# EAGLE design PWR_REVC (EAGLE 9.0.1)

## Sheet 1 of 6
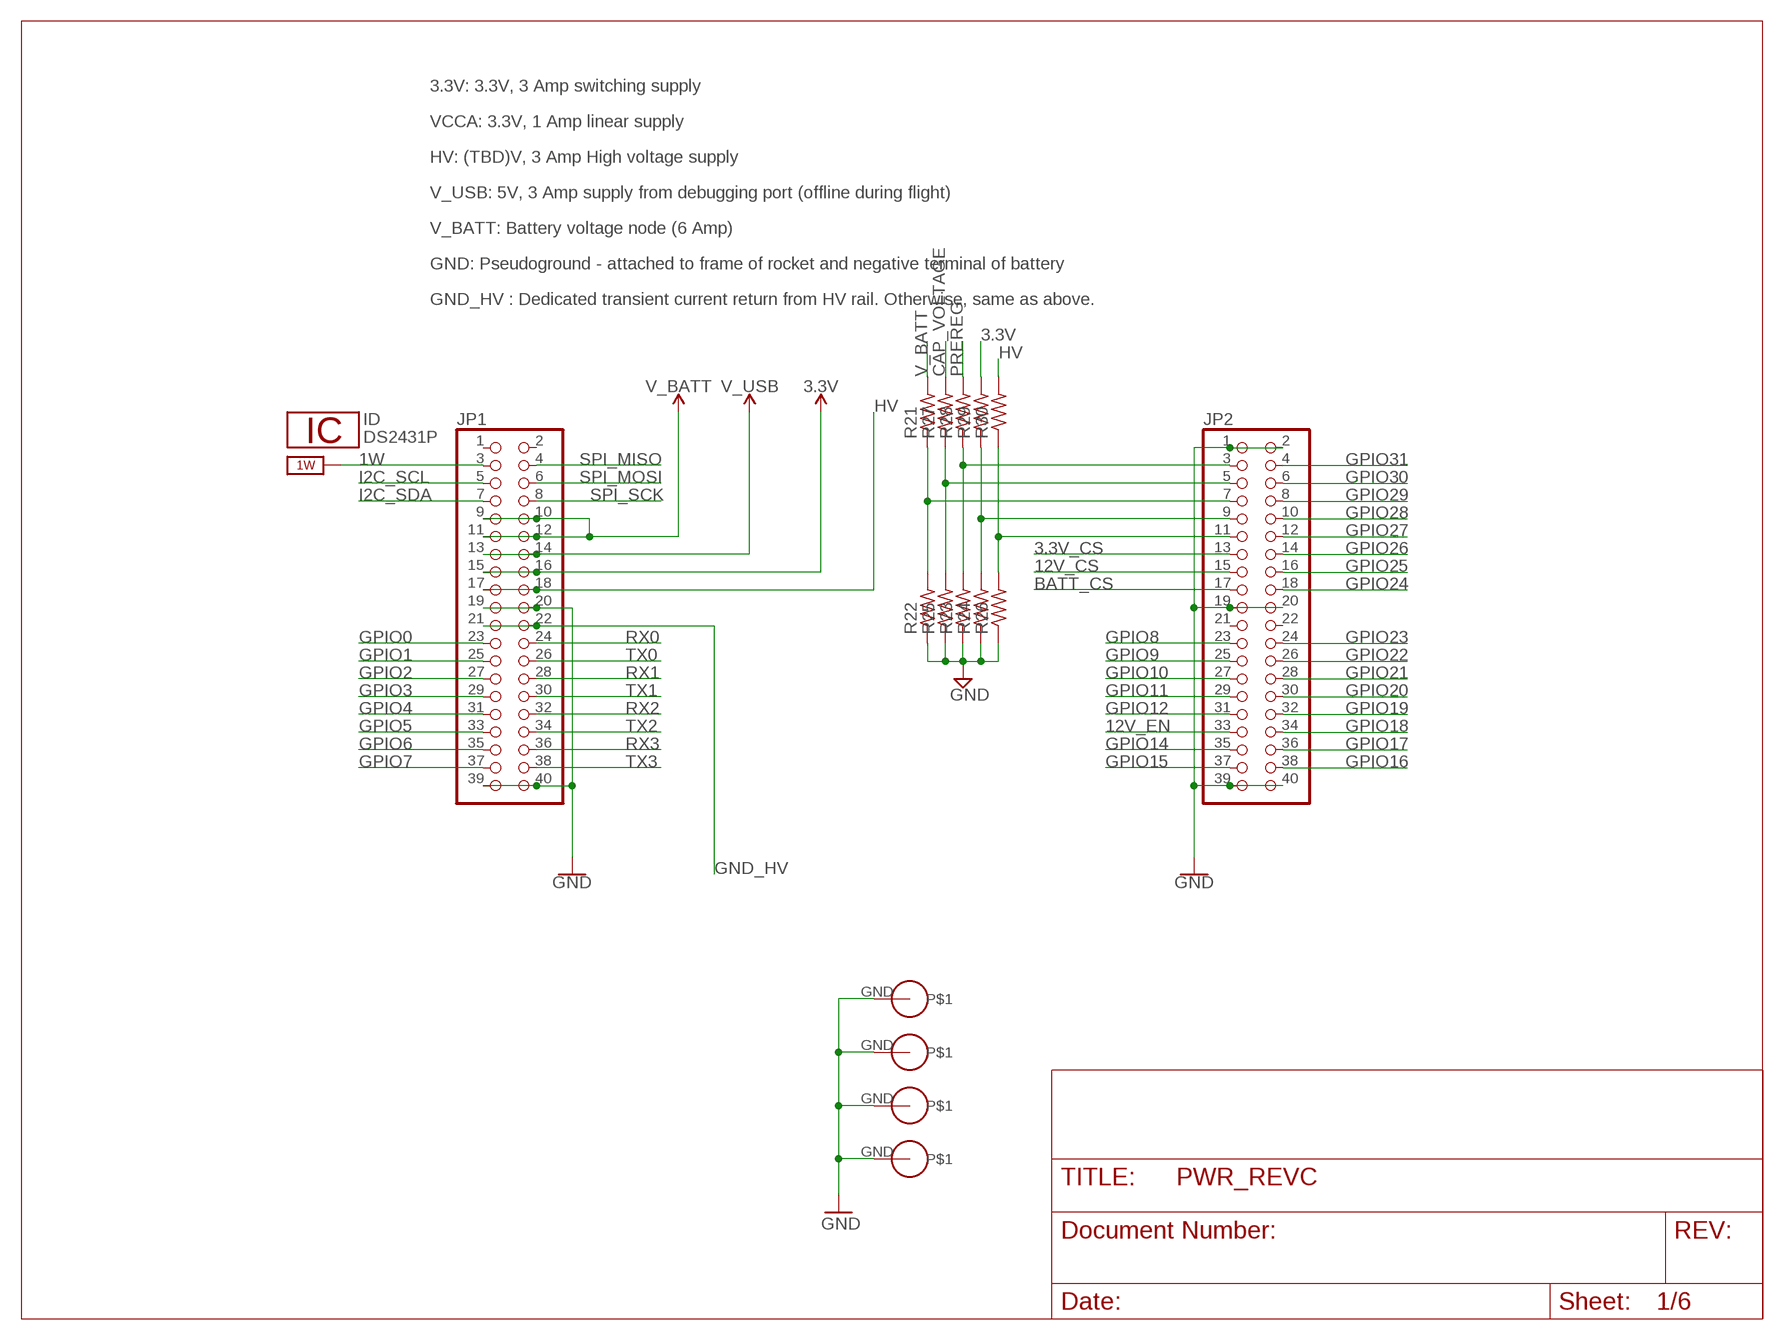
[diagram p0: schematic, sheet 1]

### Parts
ID  DS2431P  [TSOC6]
JP1  PINHD-2X20  [2X20]
JP2  PINHD-2X20  [2X20]
R21  R-US_R1206  [R1206]
R22  R-US_R1206  [R1206]
R23  R-US_R1206  [R1206]
R24  R-US_R1206  [R1206]
R25  R-US_R1206  [R1206]
R26  R-US_R1206  [R1206]
R27  R-US_R1206  [R1206]
R28  R-US_R1206  [R1206]
R29  R-US_R1206  [R1206]
R30  R-US_R1206  [R1206]
U$1  PS/104-MOUNTING-HOLE  [PC/104-MOUNTING-HOLE]
U$2  PS/104-MOUNTING-HOLE  [PC/104-MOUNTING-HOLE]
U$3  PS/104-MOUNTING-HOLE  [PC/104-MOUNTING-HOLE]
U$4  PS/104-MOUNTING-HOLE  [PC/104-MOUNTING-HOLE]

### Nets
1W: JP1.3 ; supply symbol labelled 1W_SUP
3.3V: JP1.15 JP1.16 R29.2 ; also sheet 2,6
3.3V_CS: JP2.13 ; also sheet 6
12V_CS: JP2.15 ; also sheet 6
12V_EN: JP2.33 ; also sheet 4
BATT_CS: JP2.17 ; also sheet 6
CAP_VOLTAGE: R27.2 ; also sheet 5
GND: JP1.19 JP1.20 JP1.39 JP1.40 JP2.1 JP2.2 JP2.19 JP2.20 JP2.39 JP2.40 R22.1 R23.1 R24.1 R25.1 R26.1 U$1.GND U$2.GND U$3.GND U$4.GND ; also sheet 2,3,4,5,6
GND_HV: JP1.21 JP1.22 ; also sheet 4
GPIO0: JP1.23
GPIO1: JP1.25
GPIO2: JP1.27
GPIO3: JP1.29
GPIO4: JP1.31
GPIO5: JP1.33
GPIO6: JP1.35
GPIO7: JP1.37
GPIO8: JP2.23
GPIO9: JP2.25
GPIO10: JP2.27
GPIO11: JP2.29
GPIO12: JP2.31
GPIO14: JP2.35
GPIO15: JP2.37
GPIO16: JP2.38
GPIO17: JP2.36
GPIO18: JP2.34
GPIO19: JP2.32
GPIO20: JP2.30
GPIO21: JP2.28
GPIO22: JP2.26
GPIO23: JP2.24
GPIO24: JP2.18
GPIO25: JP2.16
GPIO26: JP2.14
GPIO27: JP2.12
GPIO28: JP2.10
GPIO29: JP2.8
GPIO30: JP2.6
GPIO31: JP2.4
HV: JP1.17 JP1.18 R30.2 ; also sheet 4,6
I2C_SCL: JP1.5
I2C_SDA: JP1.7
N$28: JP2.7 R21.1 R22.2
N$30: JP2.5 R25.2 R27.1
N$31: JP2.3 R23.2 R28.1
N$32: JP2.9 R24.2 R29.1
N$33: JP2.11 R26.2 R30.1
PREREG: R28.2 ; also sheet 2,3,4,5
RX0: JP1.24
RX1: JP1.28
RX2: JP1.32
RX3: JP1.36
SPI_MISO: JP1.4
SPI_MOSI: JP1.6
SPI_SCK: JP1.8
TX0: JP1.26
TX1: JP1.30
TX2: JP1.34
TX3: JP1.38
V_BATT: JP1.9 JP1.10 JP1.11 JP1.12 R21.2 ; also sheet 3,6
V_USB: JP1.13 JP1.14
Unconnected: JP1.1 JP1.2 JP2.21 JP2.22

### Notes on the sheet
- 3.3V: 3.3V, 3 Amp switching supply
- VCCA: 3.3V, 1 Amp linear supply
- HV: (TBD)V, 3 Amp High voltage supply
- V_USB: 5V, 3 Amp supply from debugging port (offline during flight)
- V_BATT: Battery voltage node (6 Amp)
- GND: Pseudoground - attached to frame of rocket and negative terminal of battery
- GND_HV : Dedicated transient current return from HV rail. Otherwise, same as above.

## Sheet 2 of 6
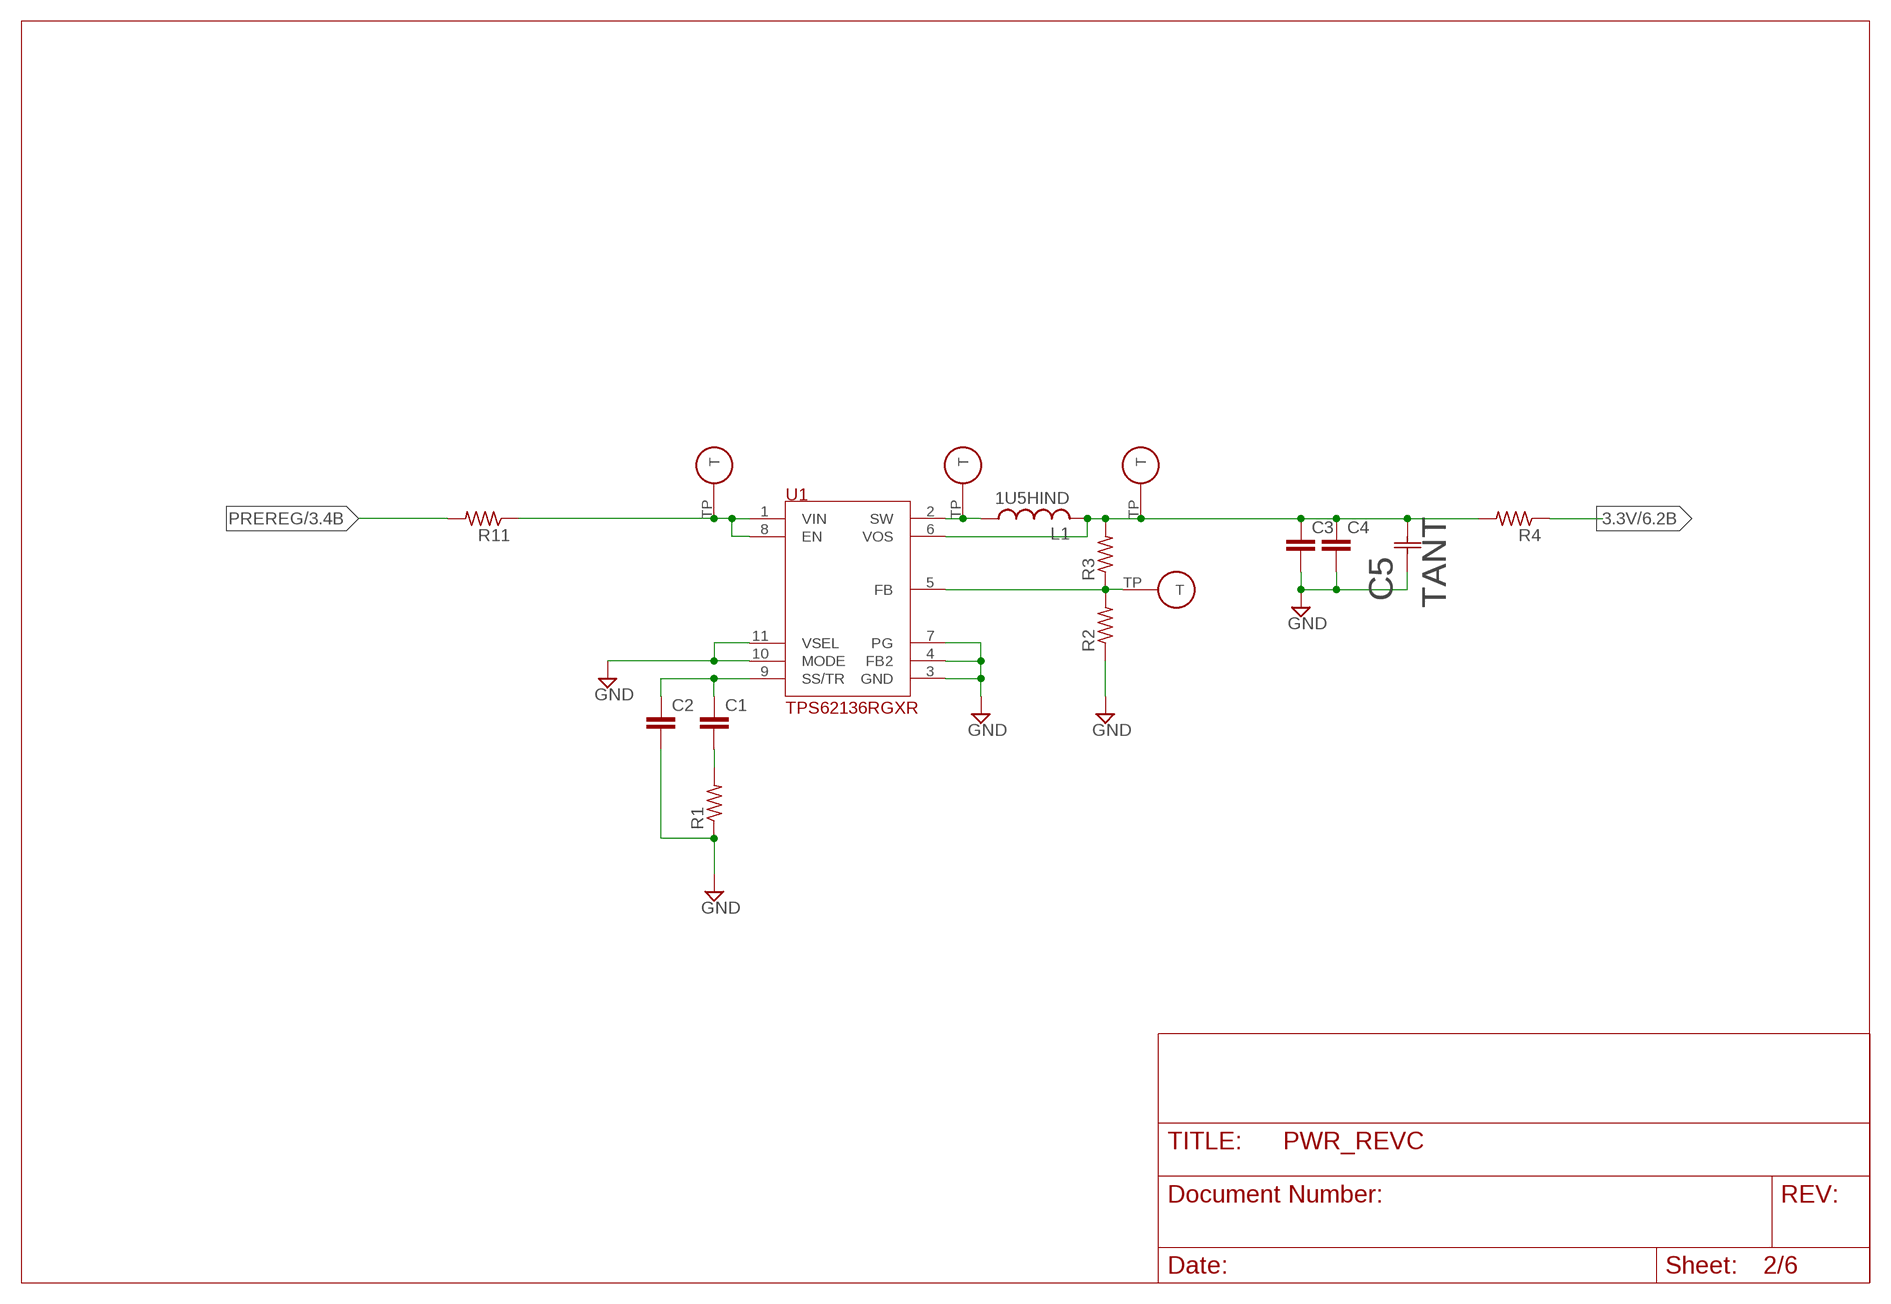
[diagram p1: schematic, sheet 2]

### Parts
C1  C-EUC0805  [C0805]
C2  C-EUC0805  [C0805]
C3  C-EUC0805  [C0805]
C4  C-EUC0805  [C0805]
C5  TANT  [CAP_593D_E]
L1  1U5HIND  [SMD_IND1U5]
R1  R-US_R1206  [R1206]
R2  R-US_R1206  [R1206]
R3  R-US_R1206  [R1206]
R4  R-US_R1206  [R1206]
R11  R-US_R1206  [R1206]
TP1  TESTPOINT  [TESTPOINT]
TP2  TESTPOINT  [TESTPOINT]
TP3  TESTPOINT  [TESTPOINT]
TP4  TESTPOINT  [TESTPOINT]
U1  TPS62136RGXR  [TPS62136RGXR]

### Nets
3.3V: R4.1 ; also sheet 1,6
GND: C2.2 C3.2 C4.2 C5.1 R1.1 R2.1 U1.3(GND) U1.4(FB2) U1.7(PG) U1.10(MODE) U1.11(VSEL) ; also sheet 1,3,4,5,6
N$6: C1.1 C2.1 U1.9(SS/TR)
N$7: C1.2 R1.2
N$8: L1.P$1 TP3.TP(T) U1.2(SW)
N$10: R11.1 TP1.TP(T) U1.1(VIN) U1.8(EN)
N$11: R2.2 R3.1 TP4.TP(T) U1.5(FB)
N$12: C3.1 C4.1 C5.2 L1.P$2 R3.2 R4.2 TP2.TP(T) U1.6(VOS) ; also sheet 6
PREREG: R11.2 ; also sheet 1,3,4,5

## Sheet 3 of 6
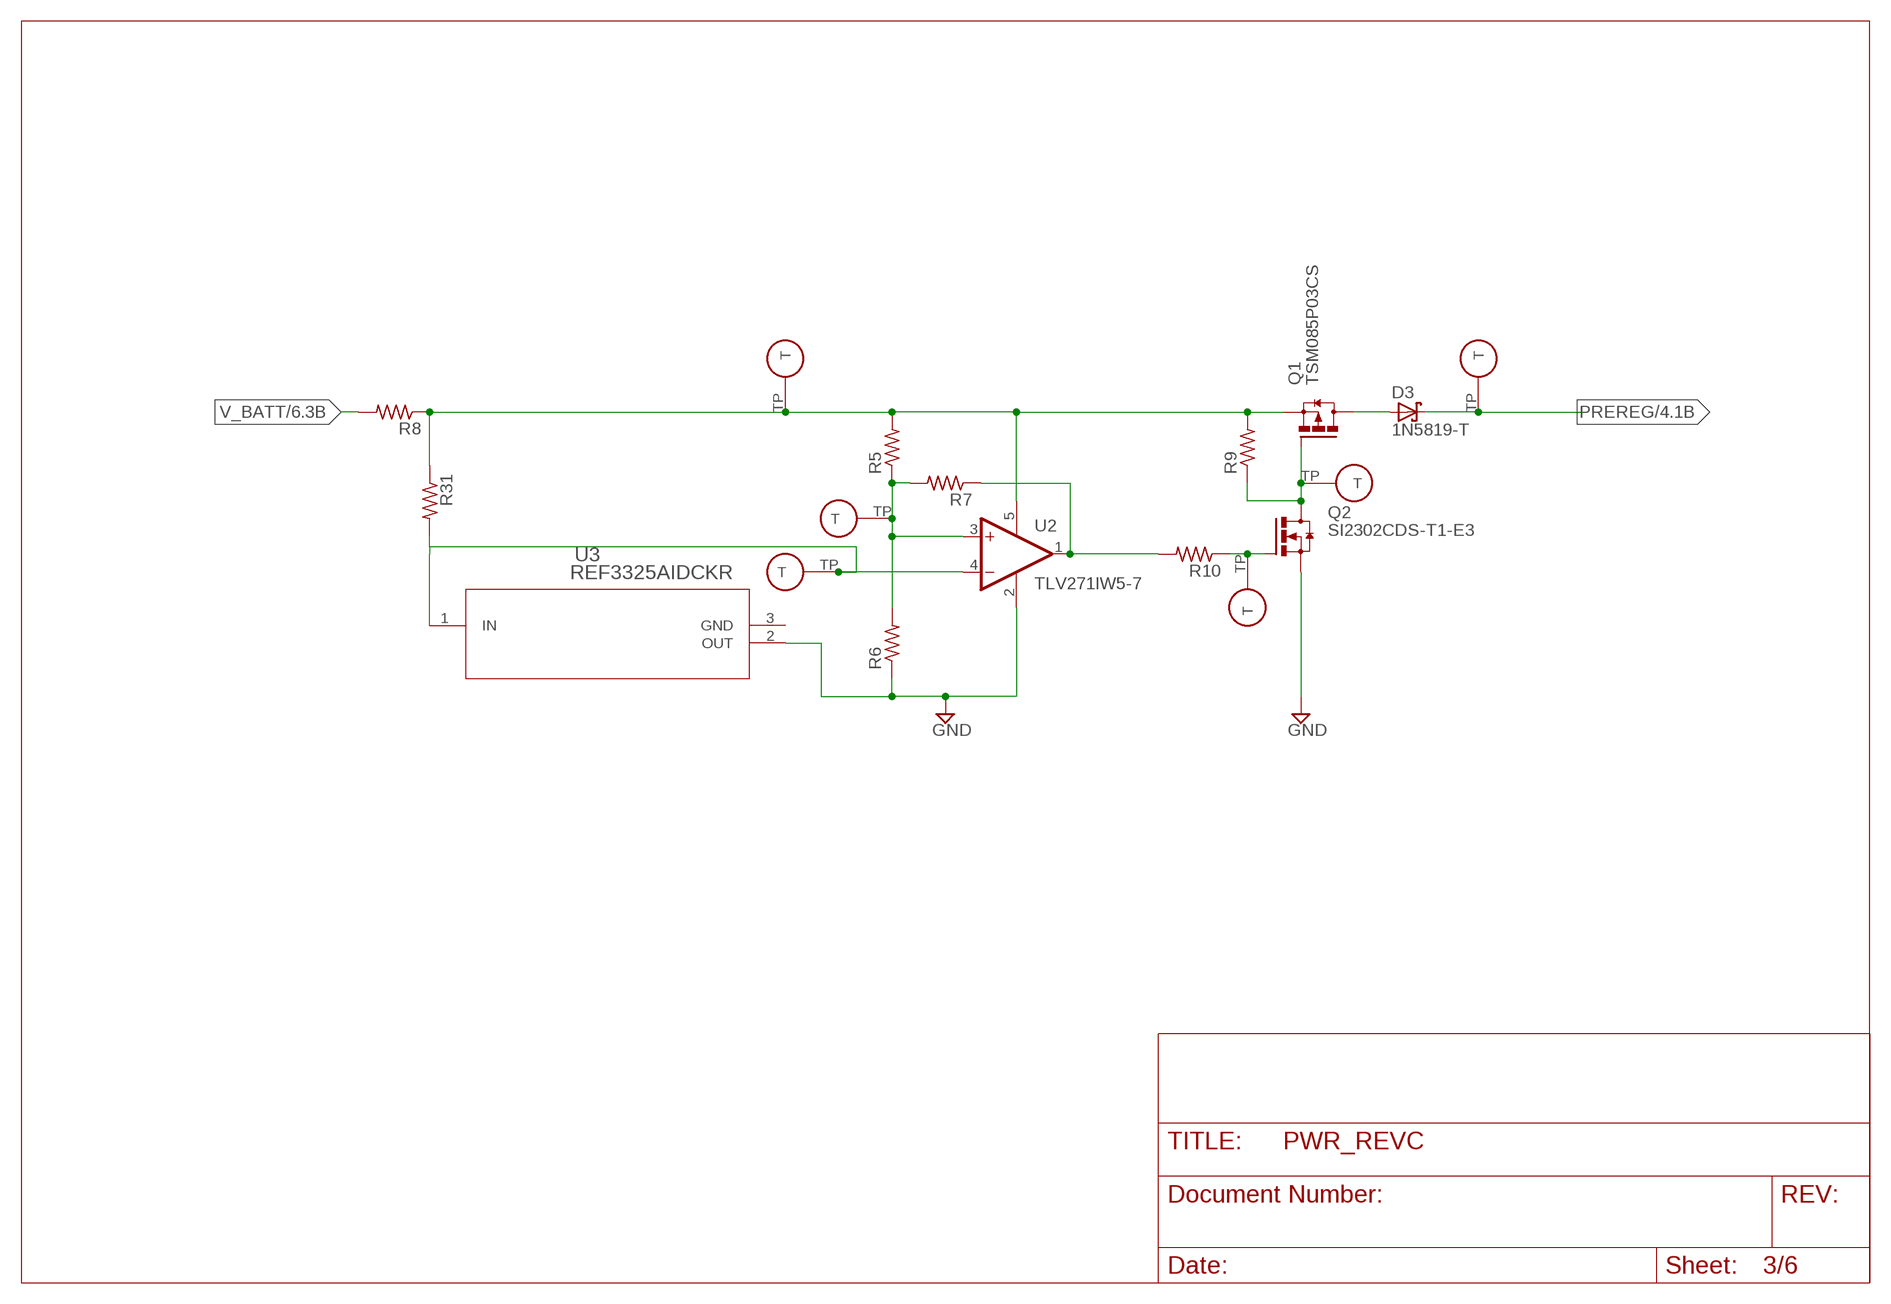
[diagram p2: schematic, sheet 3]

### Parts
D3  1N5819-T  [DO41-7.6]
Q1  TSM085P03CS  [SO08]
Q2  SI2302CDS-T1-E3  [TO-236]
R5  R-US_R1206  [R1206]
R6  R-US_R1206  [R1206]
R7  R-US_R1206  [R1206]
R8  R-US_R1206  [R1206]
R9  R-US_R1206  [R1206]
R10  R-US_R1206  [R1206]
R31  R-US_R1206  [R1206]
TP5  TESTPOINT  [TESTPOINT]
TP6  TESTPOINT  [TESTPOINT]
TP7  TESTPOINT  [TESTPOINT]
TP8  TESTPOINT  [TESTPOINT]
TP9  TESTPOINT  [TESTPOINT]
TP10  TESTPOINT  [TESTPOINT]
U2  TLV271IW5-7  [SOT25]
U3  REF3325AIDCKR  [DCK3]

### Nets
GND: Q2.2(S) R6.1 U2.2(V-) U3.2(OUT) ; also sheet 1,2,4,5,6
N$2: R5.1 R6.2 R7.2 TP7.TP(T) U2.3(+IN)
N$3: R7.1 R10.2 U2.1(OUT)
N$4: Q1.4(G) Q2.3(D) R9.1 TP9.TP(T)
N$9: R31.2 TP8.TP(T) U2.4(-IN) U3.1(IN)
N$13: Q2.1(G) R10.1 TP10.TP(T)
N$26: D3.A Q1.5(D) Q1.6(D) Q1.7(D) Q1.8(D) ; also sheet 5
N$100: Q1.1(S) Q1.2(S) Q1.3(S) R5.2 R8.1 R9.2 R31.1 TP5.TP(T) U2.5(V+) ; also sheet 6
PREREG: D3.C TP6.TP(T) ; also sheet 1,2,4,5
V_BATT: R8.2 ; also sheet 1,6

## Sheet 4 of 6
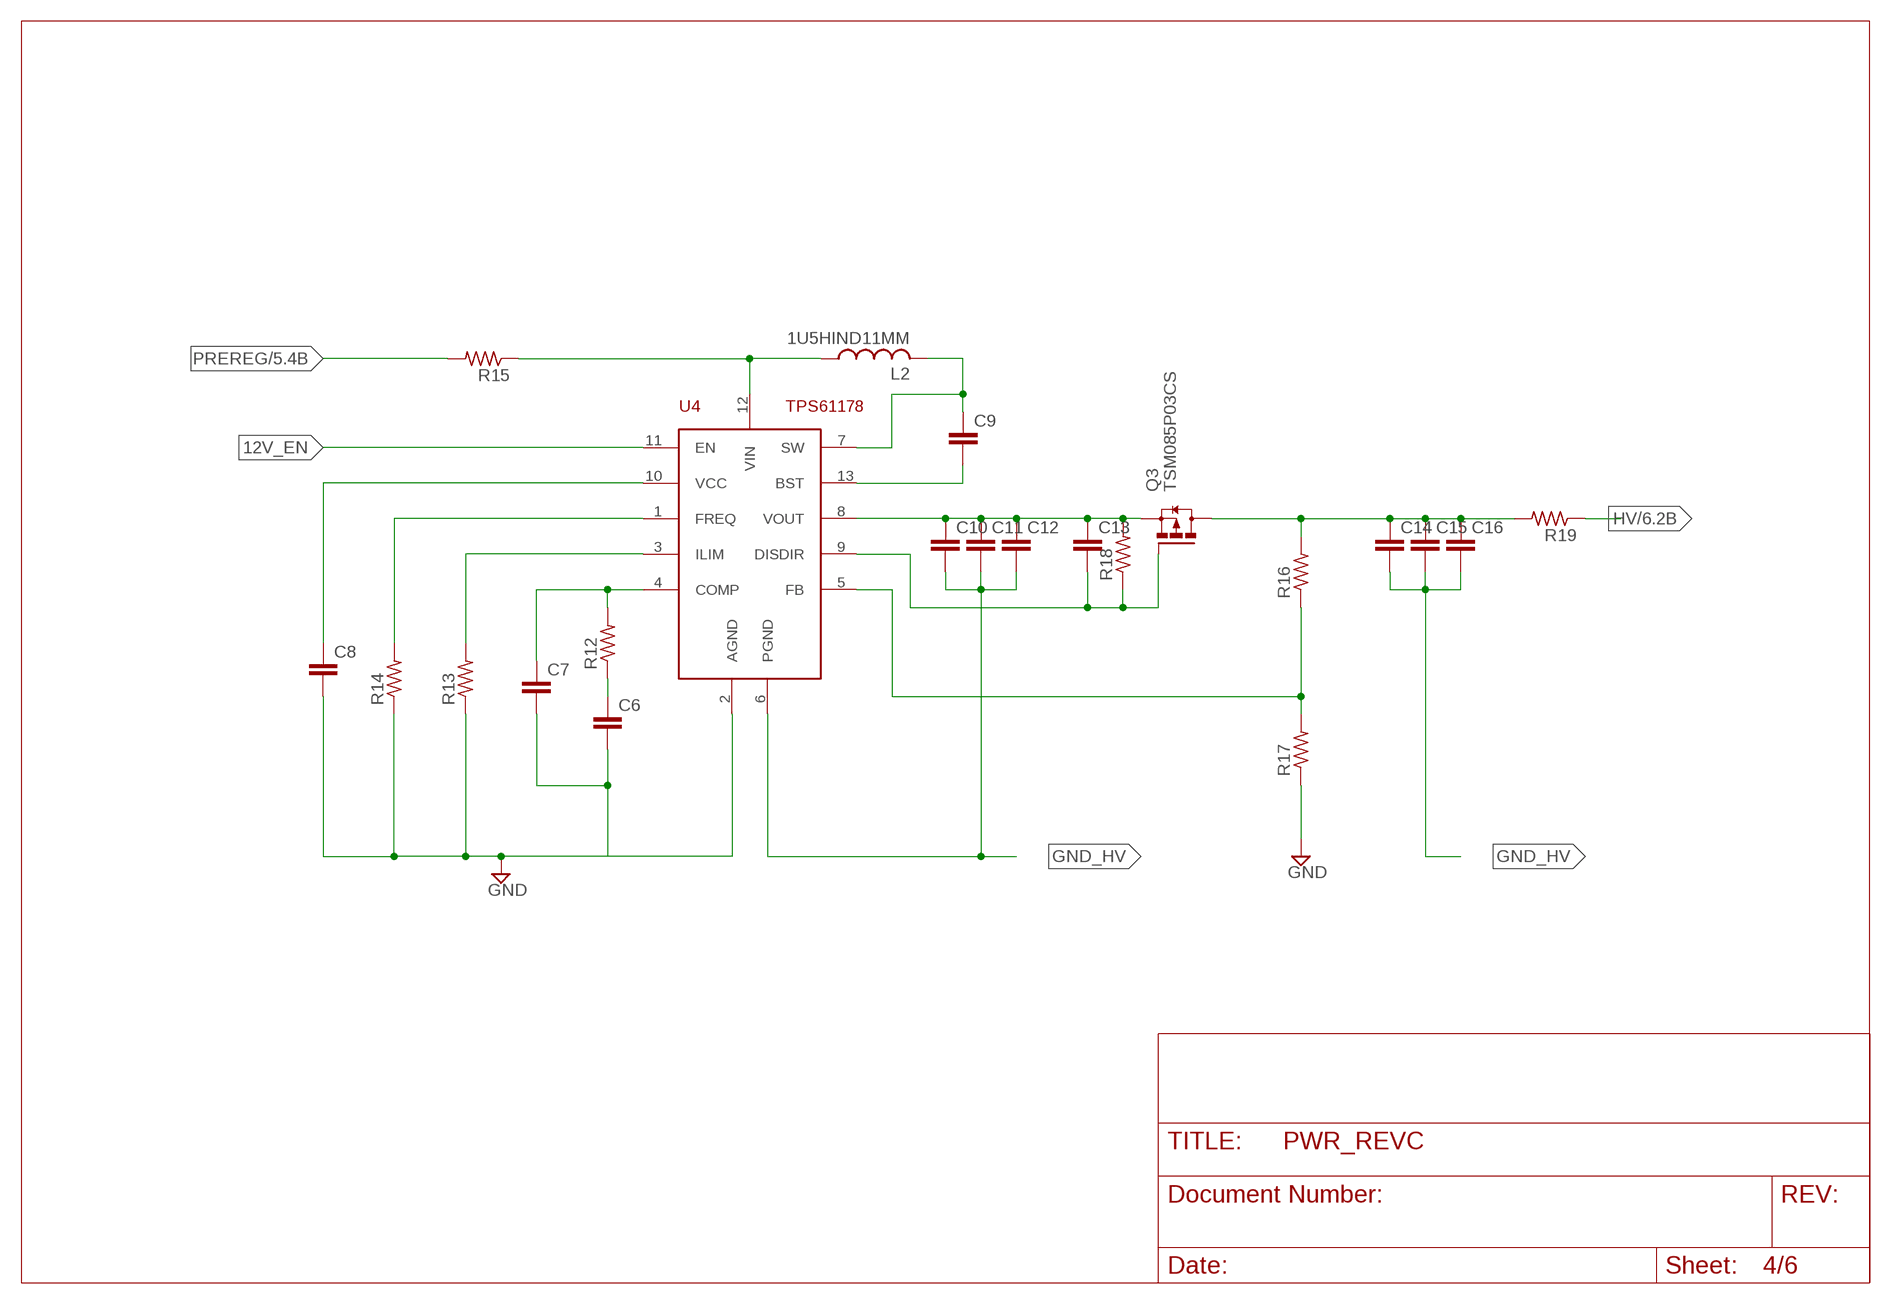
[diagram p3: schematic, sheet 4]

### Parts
C6  C-EUC0805  [C0805]
C7  C-EUC0805  [C0805]
C8  C-EUC0805  [C0805]
C9  C-EUC0805  [C0805]
C10  C-EUC0805  [C0805]
C11  C-EUC0805  [C0805]
C12  C-EUC0805  [C0805]
C13  C-EUC0805  [C0805]
C14  C-EUC0805  [C0805]
C15  C-EUC0805  [C0805]
C16  C-EUC0805  [C0805]
L2  1U5HIND11MM  [11MM]
Q3  TSM085P03CS  [SO08]
R12  R-US_R1206  [R1206]
R13  R-US_R1206  [R1206]
R14  R-US_R1206  [R1206]
R15  R-US_R1206  [R1206]
R16  R-US_R1206  [R1206]
R17  R-US_R1206  [R1206]
R18  R-US_R1206  [R1206]
R19  R-US_R1206  [R1206]
U4  TPS61178  [TPS61178]

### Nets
12V_EN: U4.11(EN) ; also sheet 1
GND: C6.2 C7.2 C8.2 R13.1 R14.1 R17.1 U4.2(AGND) ; also sheet 1,2,3,5,6
GND_HV: C10.2 C11.2 C12.2 C14.2 C15.2 C16.2 U4.6(PGND) ; also sheet 1
HV: R19.1 ; also sheet 1,6
N$1: C7.1 R12.2 U4.4(COMP)
N$14: C6.1 R12.1
N$16: R13.2 U4.3(ILIM)
N$17: R14.2 U4.1(FREQ)
N$18: L2.P$1 R15.1 U4.12(VIN)
N$19: C8.1 U4.10(VCC)
N$20: C9.2 U4.13(BST)
N$21: C9.1 L2.P$2 U4.7(SW)
N$22: C10.1 C11.1 C12.1 C13.1 Q3.1(S) Q3.2(S) Q3.3(S) R18.2 U4.8(VOUT)
N$23: C14.1 C15.1 C16.1 Q3.5(D) Q3.6(D) Q3.7(D) Q3.8(D) R16.2 R19.2 ; also sheet 6
N$24: R16.1 R17.2 U4.5(FB)
N$27: C13.2 Q3.4(G) R18.1 U4.9(DISDIR)
PREREG: R15.2 ; also sheet 1,2,3,5

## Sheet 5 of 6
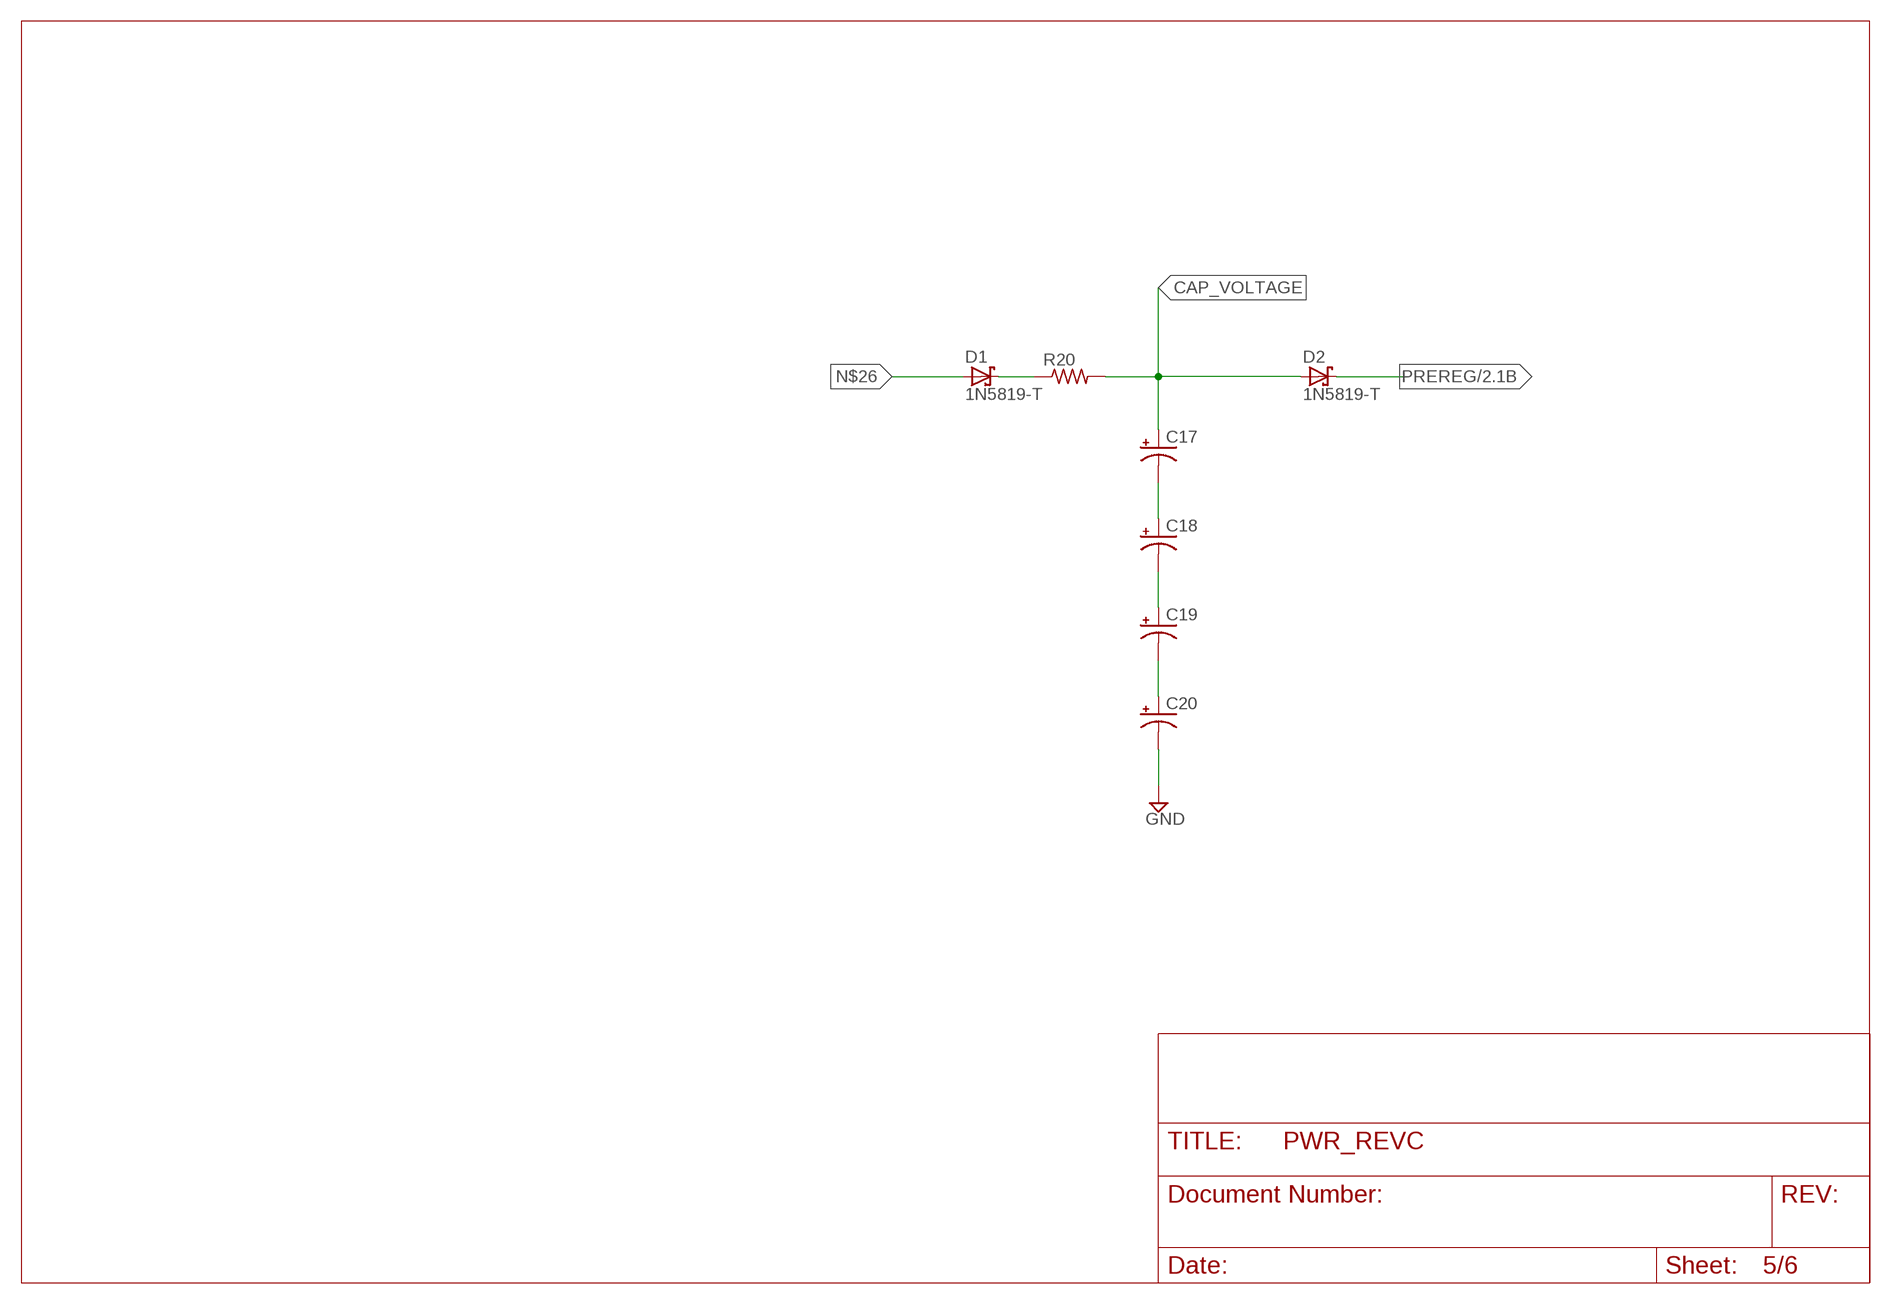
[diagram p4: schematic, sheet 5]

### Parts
C17  SUPERCAP  [SUPERCAP]
C18  SUPERCAP  [SUPERCAP]
C19  SUPERCAP  [SUPERCAP]
C20  SUPERCAP  [SUPERCAP]
D1  1N5819-T  [DO41-7.6]
D2  1N5819-T  [DO41-7.6]
R20  R-US_0207/10  [0207/10]

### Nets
CAP_VOLTAGE: C17.+ D2.A R20.2 ; also sheet 1
GND: C20.- ; also sheet 1,2,3,4,6
N$5: C19.- C20.+
N$15: C18.- C19.+
N$25: C17.- C18.+
N$26: D1.A ; also sheet 3
N$29: D1.C R20.1
PREREG: D2.C ; also sheet 1,2,3,4

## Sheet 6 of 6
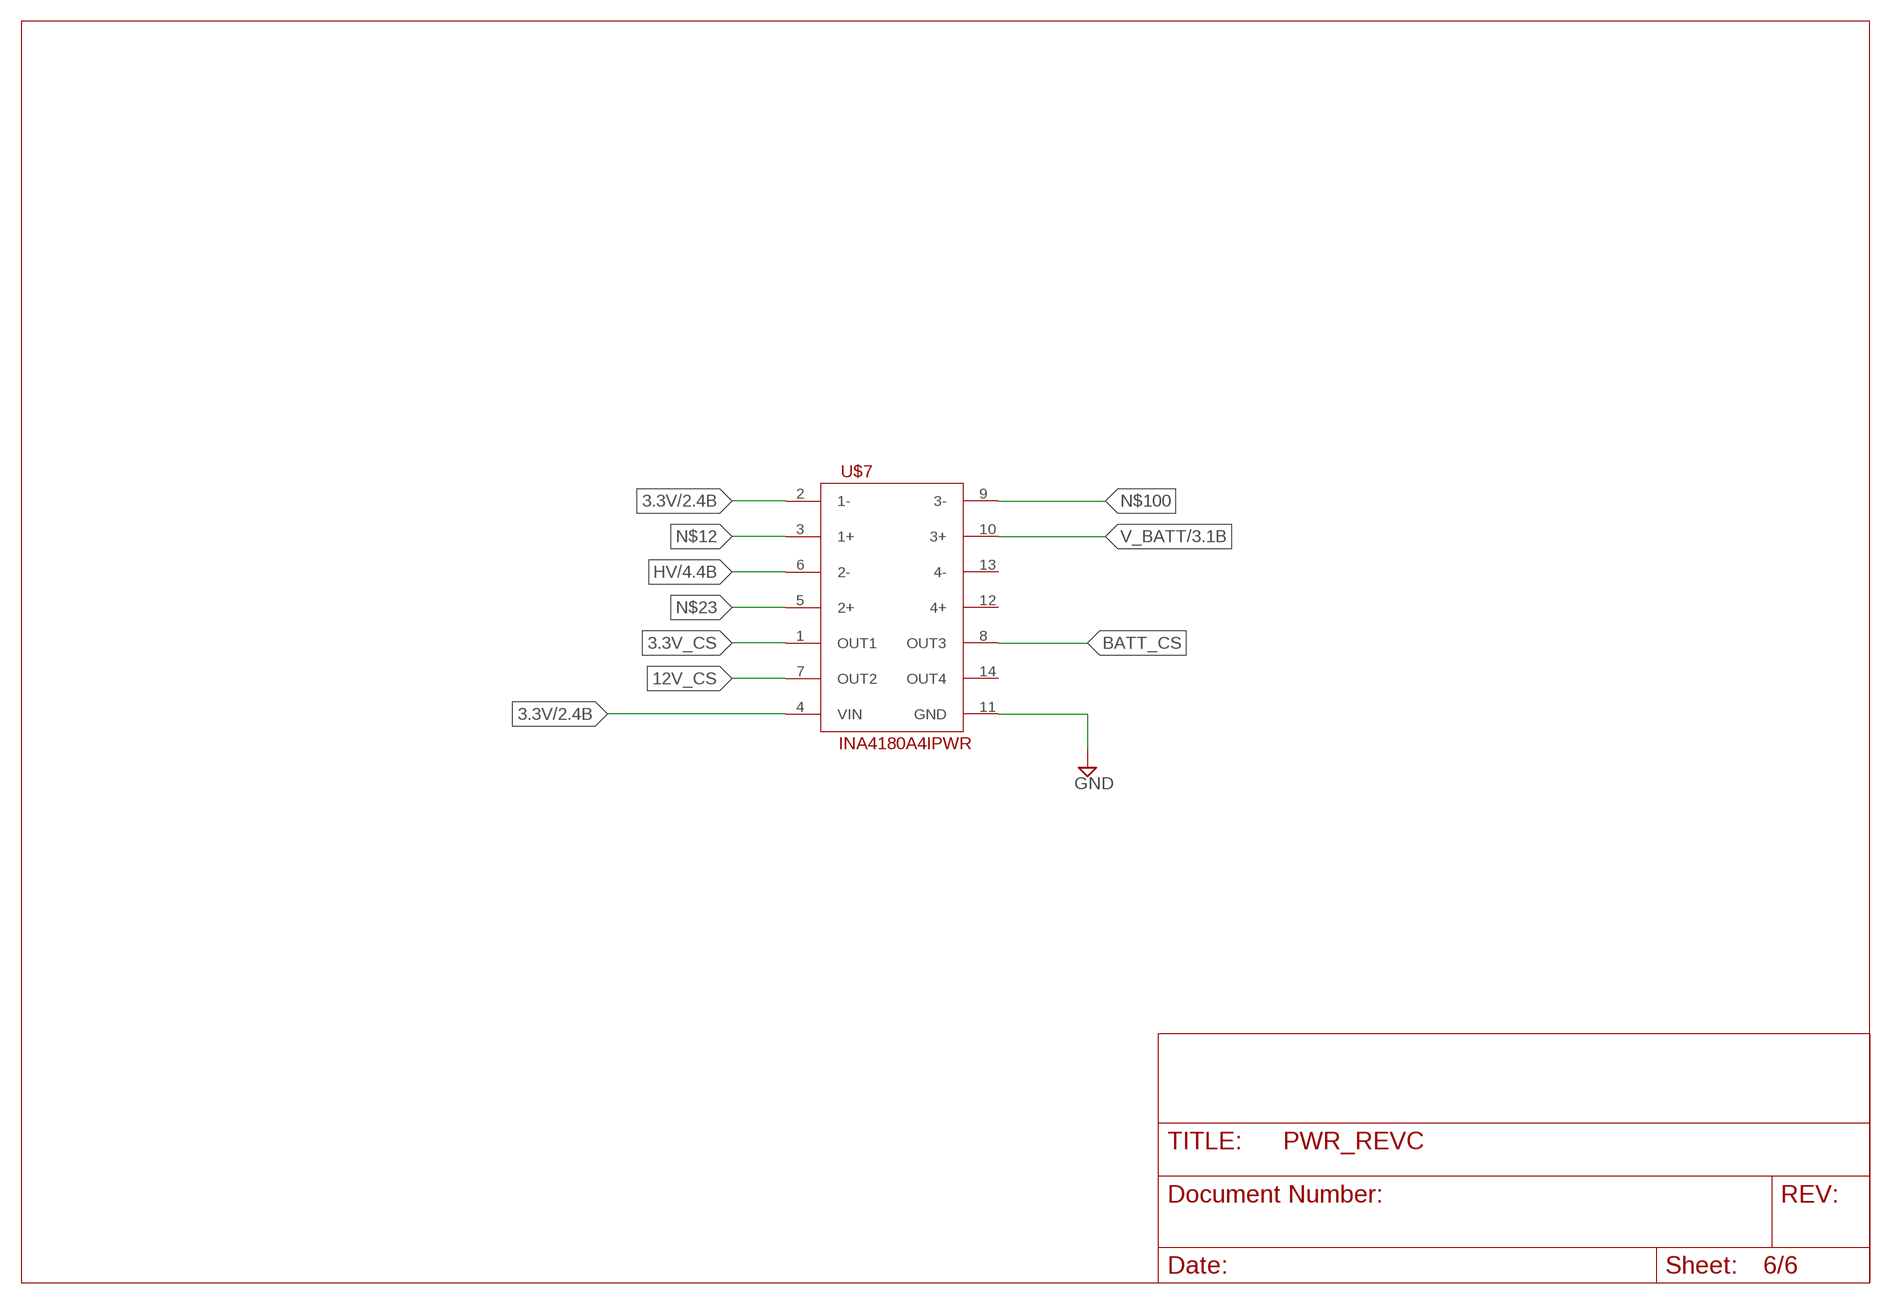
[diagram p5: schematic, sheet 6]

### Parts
U$7  INA4180A4IPWR  [TSSOP14]

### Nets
3.3V: U$7.2(1-) U$7.4(VIN) ; also sheet 1,2
3.3V_CS: U$7.1(OUT1) ; also sheet 1
12V_CS: U$7.7(OUT2) ; also sheet 1
BATT_CS: U$7.8(OUT3) ; also sheet 1
GND: U$7.11(GND) ; also sheet 1,2,3,4,5
HV: U$7.6(2-) ; also sheet 1,4
N$12: U$7.3(1+) ; also sheet 2
N$23: U$7.5(2+) ; also sheet 4
N$100: U$7.9(3-) ; also sheet 3
V_BATT: U$7.10(3+) ; also sheet 1,3
Unconnected: U$7.12(4+) U$7.13(4-) U$7.14(OUT4)

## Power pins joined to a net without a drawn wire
1W: ID.2(1W)
GND: ID.1(GND) U3.3(GND)

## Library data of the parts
C1-C4 C6-C16 = rcl:C-EU: CAPACITOR, European symbol; SPICEPREFIX: C
C5 = CU inSpace 2019 Parts:TANT
C17-C20 = CU inSpace 2019 Parts:SUPERCAP
D1-D3 = diode:1N581*: 1.0A SCHOTTKY BARRIER RECTIFIER
ID = 1wire:DS2431: 1024-Bit EEPROM
JP1 JP2 = pinhead:PINHD-2X20: PIN HEADER
L1 L2 = CU inSpace 2019 Parts:1U5HIND
Q1 Q3 = LibFaradayGen:TSM085P03CS: 30V 34A Vth -1.5V
Q2 = LibFaradayGen:SI2302CDS-T1-E3
R1-R31 = rcl:R-US_: RESISTOR, American symbol; SPICEPREFIX: R
TP1-TP10 = CU inSpace 2019 Parts:TESTPOINT
U1 = CU inSpace 2019 Parts:TPS62136RGXR
U2 = CU inSpace 2019 Parts:TLV271IW5-7; MANUFACTURER_PART_NUMBER: TLV271IW57; VENDOR: Diodes Inc
U3 = CU inSpace 2019 Parts:REF3325AIDCKR; MANUFACTURER_PART_NUMBER: REF3325AIDCKR; VENDOR: Texas Instruments
U4 = CU inSpace 2019 Parts:TPS61178
U$1-U$4 = CU inSpace 2019 Parts:PS/104-MOUNTING-HOLE: Mounting hole for PC/104 board.
U$7 = CU inSpace 2019 Parts:INA4180A4IPWR

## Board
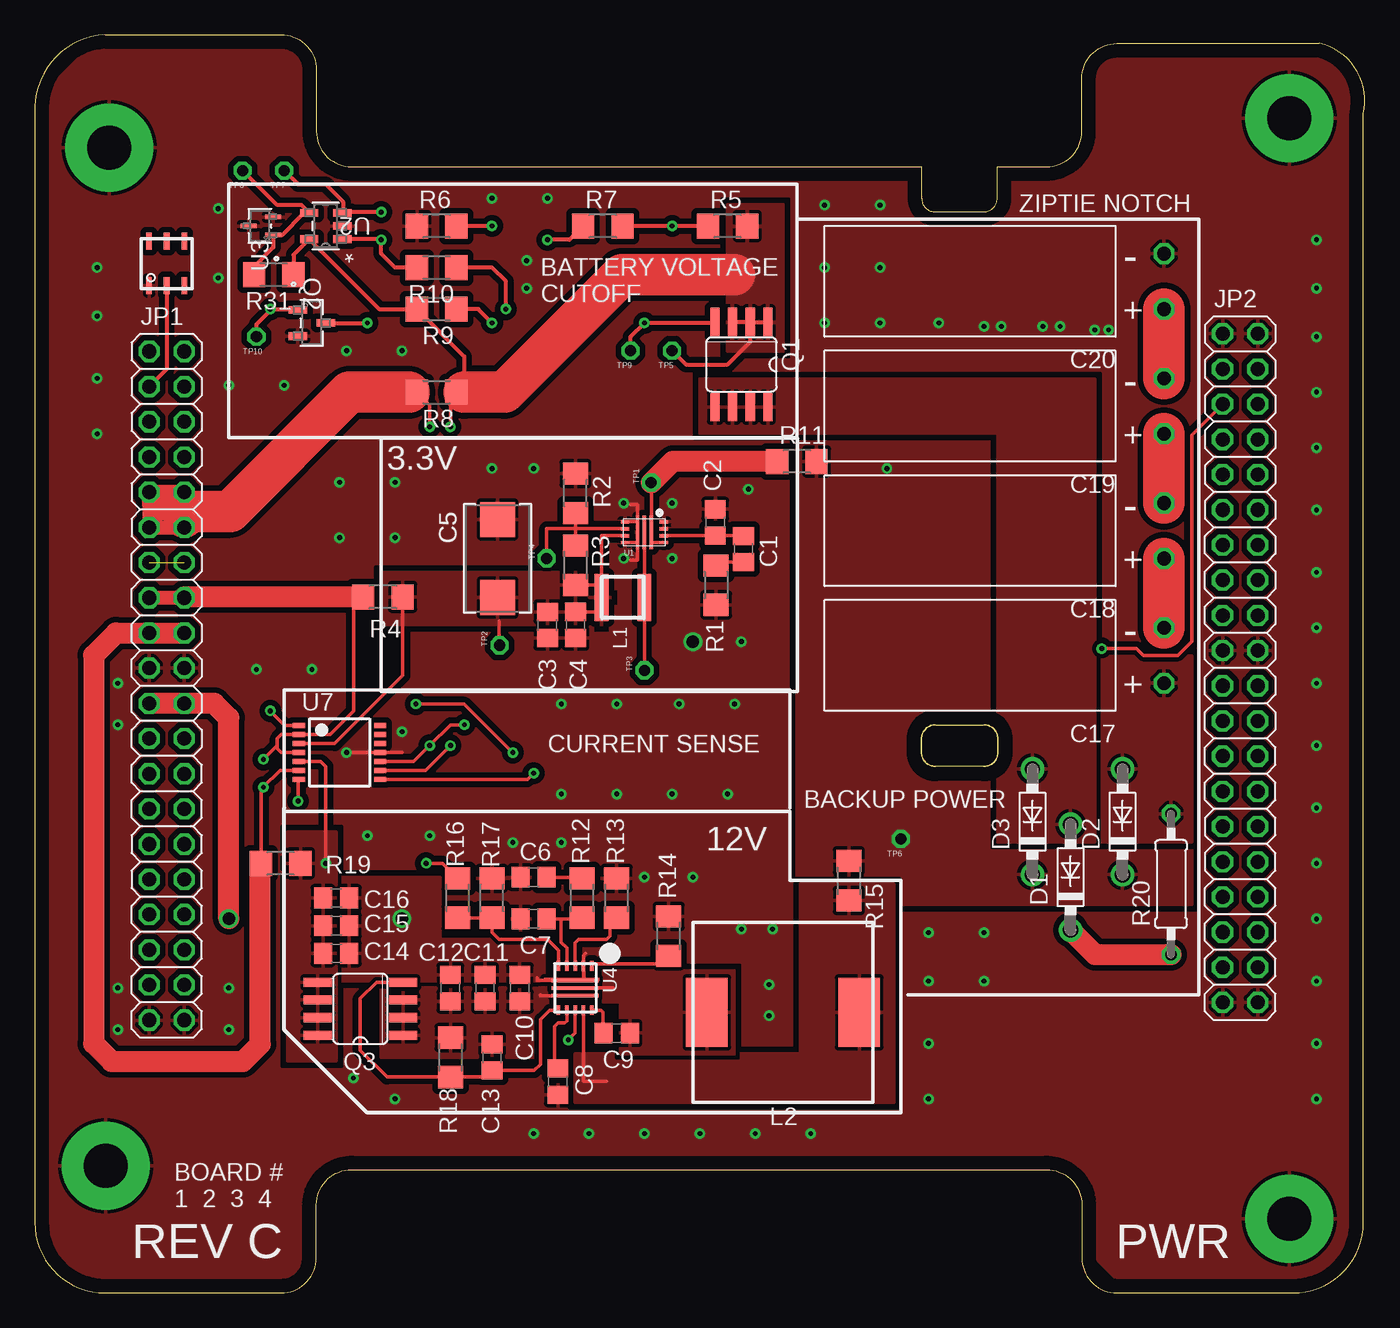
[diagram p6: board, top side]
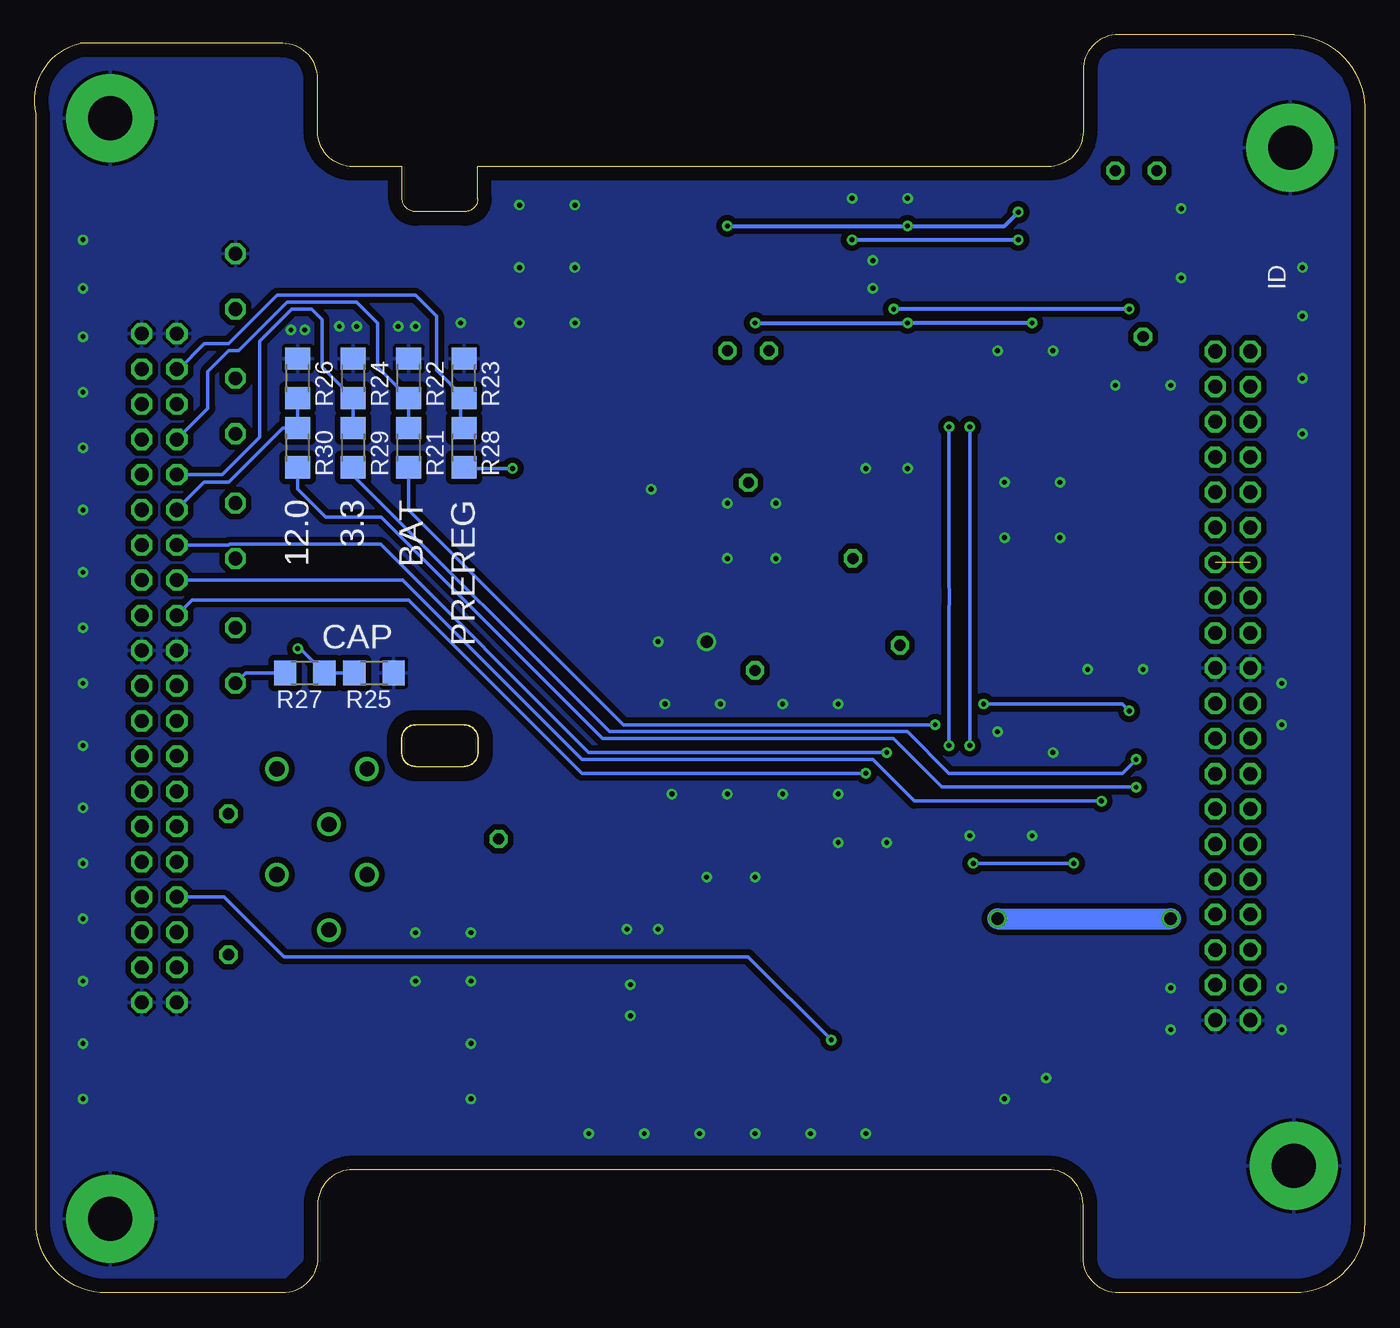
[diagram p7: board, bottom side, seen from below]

Size 96 x 90.81 mm. Coordinates in mm from the lower left corner, seen from the top.
Outline: 5.09,0 17.79,0 arc90 20.33,2.54 20.33,6.35 arc-90 22.87,8.89 73.03,8.89 arc-90 75.57,6.35 75.57,2.54 arc90 78.11,0 90.81,0 arc90 95.89,5.08 95.89,85.09 arc90 92.72,90.17 78.11,90.17 arc90 75.57,87.63 75.57,83.82 arc-90 73.03,81.28 69.48,81.28 69.48,78.99 arc-90 68.51,78.03 65.01,78.03 arc-93 64.01,78.97 64.01,81.28 22.87,81.28 arc-90 20.33,83.82 20.33,88.27 arc90 17.79,90.81 5.09,90.81 arc90 0.01,85.09 0.01,5.08 arc90 5.09,0
Outline: 65.01,41 68.51,41 arc-90 69.51,40 69.51,39 arc-90 68.51,38 65.01,38 arc-90 64.01,39 64.01,40 arc-90 65.01,41
Copper layers (1*16): Top 0.035mm / dielectric 1.5mm / Bottom 0.035mm
Design rules "default": minimum track width 6mil, minimum drill 0.35mm, track to track 6mil, track to pad 6mil, pad to pad 6mil, via to via 6mil, smd to smd 6mil, copper to edge 40mil, drill to drill 6mil, minimum pad ring 10mil, minimum via ring 8mil, stop-mask expansion 4mil, vias tented up to drill 0mil, thermal gap 10mil

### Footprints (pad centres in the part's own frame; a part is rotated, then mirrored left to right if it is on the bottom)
C0805 = smd 1.3 x 1.5: 1 -0.95,0; 2 0.95,0
CAP_593D_E = smd 2.54 x 2.515: 1 -2.819,0; 2 2.819,0
SUPERCAP = drill 1 octagon: + -3.5,2; - -3.5,-2
DO41-7.6 = drill 1.1 pad 1.7: A 3.81,0; C -3.81,0
TSOC6 = smd 0.406 x 1.219: 1 -1.27,-1.6; 2 0,-1.6; 3 1.27,-1.6; 4 1.27,1.6; 5 0,1.6; 6 -1.27,1.6
2X20 = drill 1.016 octagon: 1 -24.13,-1.27; 2 -24.13,1.27; 3 -21.59,-1.27; 4 -21.59,1.27; 5 -19.05,-1.27; 6 -19.05,1.27; 7 -16.51,-1.27; 8 -16.51,1.27; 9 -13.97,-1.27; 10 -13.97,1.27; 11 -11.43,-1.27; 12 -11.43,1.27; 13 -8.89,-1.27; 14 -8.89,1.27; 15 -6.35,-1.27; 16 -6.35,1.27; 17 -3.81,-1.27; 18 -3.81,1.27; 19 -1.27,-1.27; 20 -1.27,1.27; 21 1.27,-1.27; 22 1.27,1.27; 23 3.81,-1.27; 24 3.81,1.27; 25 6.35,-1.27; 26 6.35,1.27; 27 8.89,-1.27; 28 8.89,1.27; 29 11.43,-1.27; 30 11.43,1.27; 31 13.97,-1.27; 32 13.97,1.27; 33 16.51,-1.27; 34 16.51,1.27; 35 19.05,-1.27; 36 19.05,1.27; 37 21.59,-1.27; 38 21.59,1.27; 39 24.13,-1.27; 40 24.13,1.27
SMD_IND1U5 = smd 1 x 3.4: P$1 1.55,0; P$2 -1.55,0
11MM = smd 3 x 5: P$1 5.5,0; P$2 -5.5,0
SO08 = smd 0.66 x 2.032: 1 -1.905,-3.073; 2 -0.635,-3.073; 3 0.635,-3.073; 4 1.905,-3.073; 5 1.905,3.073; 6 0.635,3.073; 7 -0.635,3.073; 8 -1.905,3.073
TO-236 = smd 0.559 x 1.321: 1 -0.95,-1.016; 2 0.95,-1.016; 3 0,1.016
R1206 = smd 1.6 x 1.803: 1 -1.422,0; 2 1.422,0
0207/10 = drill 0.813 octagon: 1 -5.08,0; 2 5.08,0
TESTPOINT = drill 0.8 octagon: TP 0,0
TPS62136RGXR = smd 2.4 x 0.25: 1 0,0.5; 2 0,0; 3 0,-0.5 | smd 0.25 x 0.6: 4 -0.75,-1.4; 5 -0.25,-1.4; 6 0.25,-1.4; 7 0.75,-1.4; 8 0.75,1.4; 9 0.25,1.4; 10 -0.25,1.4; 11 -0.75,1.4
SOT25 = smd 1.311 x 0.551: 1 -1.2,0.95; 2 -1.2,0; 3 -1.2,-0.95; 4 1.2,-0.95; 5 1.2,0.95
DCK3 = smd 0.356 x 1.168: 1 -0.65,-0.965; 2 0.65,-0.965; 3 0,0.819
TPS61178 = smd 0.7 x 0.25: 1 -1.6,1.2; 2 -1.6,0.6; 3 -1.6,0; 4 -1.6,-0.6; 5 -1.6,-1.2; 9 1.6,-1.2; 10 1.6,-0.6; 11 1.6,0; 12 1.6,0.6; 13 1.6,1.2 | smd 0.25 x 3.4: 6 -0.55,0; 7 0,0; 8 0.55,0
PC/104-MOUNTING-HOLE = drill 3.175 pad 6.35: GND 0,0
TSSOP14 = smd 0.35 x 0.9: 1 -1.95,-2.925; 2 -1.3,-2.925; 3 -0.65,-2.925; 4 0,-2.925; 5 0.65,-2.925; 6 1.3,-2.925; 7 1.95,-2.925; 8 1.95,2.925; 9 1.3,2.925; 10 0.65,2.925; 11 0,2.925; 12 -0.65,2.925; 13 -1.3,2.925; 14 -1.95,2.925

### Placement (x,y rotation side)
C1  51.16,53.69 270 top
C2  49.12,55.6 90 top
C3  37.01,48.2 270 top
C4  39.03,48.2 270 top
C5  33.41,53 270 top
C6  36.01,30 180 top
C7  36.01,27 180 top
C8  37.76,15.25 270 top
C9  42.01,18.75 180 top
C10  35.01,22 90 top
C11  32.51,22 90 top
C12  30.01,22 90 top
C13  33.01,17 270 top
C14  21.76,24.5 0 top
C15  21.76,26.5 0 top
C16  21.76,28.5 0 top
C17  78.01,46 180 top
C18  78.01,55 180 top
C19  78.01,64 180 top
C20  78.01,73 180 top
D1  74.76,30 90 top
D2  78.51,34 90 top
D3  72.01,34 90 top
ID  9.53,74.3 0 top
JP1  9.53,43.81 270 top
JP2  87,45.09 270 top
L1  42.45,50.19 0 top
L2  54.01,20.25 0 top
Q1  51.01,67 180 top
Q2  20.01,70 270 top
Q3  23.51,20.5 90 top
R1  49.18,51.08 90 top
R2  39.03,57.7 270 top
R3  39.04,52.5 270 top
R4  25.13,50.23 0 top
R5  50.01,77 0 top
R6  29.01,77 0 top
R7  41.01,77 0 top
R8  29.01,65 180 top
R9  29.01,71 180 top
R10  29.01,74 180 top
R11  55.01,60 0 top
R12  39.51,28.5 270 top
R13  42.01,28.5 270 top
R14  45.76,25.75 270 top
R15  58.76,29.75 90 top
R16  30.51,28.5 90 top
R17  33.01,28.5 270 top
R18  30.01,17 90 top
R19  17.76,31 0 top
R20  82.01,29.5 90 top
R21  69.01,61 270 bottom
R22  69.01,66 270 bottom
R23  65.01,66 270 bottom
R24  73.01,66 270 bottom
R25  71.51,44.75 180 bottom
R26  77.01,66 270 bottom
R27  76.51,44.75 180 bottom
R28  65.01,61 270 bottom
R29  73.01,61 270 bottom
R30  77.01,61 270 bottom
R31  17.26,73.5 180 top
TP1  44.5,58.48 270 top
TP2  33.54,46.74 270 top
TP3  44,44.93 270 top
TP4  36.96,53.01 270 top
TP5  46.01,68 0 top
TP6  62.51,32.75 0 top
TP7  18.01,81 0 top
TP8  15.01,81 0 top
TP9  43.01,68 0 top
TP10  16.01,69 0 top
U1  44.01,54.9 270 top
U2  21.01,77 180 top
U3  16.26,77 90 top
U4  39.01,22 270 top
U$1  5.37,82.65 0 top
U$2  90.56,84.79 0 top
U$3  5.14,9.17 0 top
U$4  90.56,5.36 0 top
U$7  22.01,39 270 top

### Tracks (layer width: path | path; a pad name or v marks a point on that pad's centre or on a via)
1W
  Top 0.305: ID.2 9.53,66.67 JP1.3
3.3V  (via drill 0.35)
  Top 0.254: R4.1 23.01,49.52 23.01,42 21.31,40.3 U$7.2 17.81,40.3 17.51,40 17.51,39.5 | U$7.4 17.81,39 17.51,39.3 17.51,39.5 | v16.51,38.5 17.51,39.5
  Top 1.016: 10.8,50.13 JP1.16 JP1.15
  Top 1.5: R4.1 10.8,50.23 JP1.16
  Bottom 0.254: v16.51,38.5 17.51,37.5 30.01,37.5 33.01,40.5 54.51,40.5 73.01,59 R29.2
3.3V_CS  (via drill 0.35)
  Top 0.254: v34.51,39 31.01,42.5 v27.51,42.5 | v17.01,42 18.06,40.95 U$7.1
  Bottom 0.254: JP2.13 81.99,53.98 81.93,54.03 71.04,54.03 56.01,39 v34.51,39 | v27.51,42.5 17.51,42.5 v17.01,42
12V_CS  (via drill 0.35)
  Top 0.254: U$7.7 19.01,36.98 v19.01,35.5
  Bottom 0.254: v19.01,35.5 32.51,35.5 35.51,38.5 56.51,38.5 69.44,51.44 JP2.15
12V_EN  (via drill 0.35)
  Top 0.254: U4.11 39.01,18.75 v38.51,18.25
  Bottom 0.254: JP2.33 82.33,28.57 78.01,24.25 44.51,24.25 v38.51,18.25
BATT_CS  (via drill 0.35)
  Top 0.254: U$7.8 35.56,37.05 v36.01,37.5
  Bottom 0.254: v36.01,37.5 56.51,37.5 69.01,50 84.63,50 JP2.17
CAP_VOLTAGE
  Bottom 0.254: 82.01,44 C17.+ 80.76,44.75 R27.2
  pour Top (isolate 0.305, rank 2): 76.51,32.5 76.51,46 83.51,46 83.51,32.5
GND  (via drill 0.35, 0.9)
  Top 0.254: U1.4 43.51,55.65 U1.3 | U1.3 43.51,56.9 43.01,56.9 | U1.3 43.51,52.9 43.01,52.9 | U1.7 43.51,54.15 U1.3 | U4.2 39.61,24.35 39.76,24.5 | 26.51,39 U$7.11 v22.51,39
  other vias: 38.01,42.5 42.01,42.5 33.01,59.5 36.01,59.5 22.01,54.5 26.01,54.5 22.01,58.5 26.01,58.5 64.51,26 68.51,26 64.51,22.5 68.51,22.5 64.51,18 64.51,14 46.51,42.5 50.51,42.5 46.01,36 50.01,36 38.01,36 42.01,36 35.51,72.5 35.51,74.5 22.51,68 26.51,68 14.01,65.5 18.01,65.5 33.01,79 37.01,79 57.01,78.5 61.01,78.5 57.01,74 61.01,74 57.01,70 61.01,70 65.26,70 69.76,69.75 74.01,69.75 77.51,69.5 52.01,11.5 56.01,11.5 44.01,11.5 48.01,11.5 36.01,11.5 40.01,11.5 23.01,15.5 26.01,14 44.01,30 47.51,30 34.51,32.5 38.01,32.5 24.01,33 28.51,33 51.51,58 47.51,47 51.01,47 42.51,53 46.01,53 42.51,57 46.01,57 26.51,40.5 16.01,45 20.01,45 92.51,44 92.51,39.5 92.51,35 92.51,31 92.51,27 92.51,22.5 92.51,18 92.51,14 92.51,61 92.51,56.5 92.51,52 92.51,48 92.51,76 92.51,72.5 92.51,69 92.51,65 4.51,74 4.51,70.5 4.51,66 4.51,62 6.01,44 6.01,41 14.01,19 14.01,22 6.01,22 6.01,19 13.26,73.25 13.26,78.25 76.51,69.5 72.76,69.75 68.51,69.75 51.01,26.25 53.26,26.25 53.01,22.25 53.01,20
  pour Top (isolate 0.406, rank 6): 25.01,9 21.01,9 20.01,8 20.01,2 18.01,0 4.01,0 1.01,3 0.01,4 0.01,7 0.01,86 5.01,91 18.01,91 20.01,89 20.01,83 22.01,81 23.01,81 74.01,81 76.01,83 76.01,88 78.01,90 93.01,90 95.01,88 96.01,87 96.01,82 96.01,3 93.01,0 79.01,0 76.01,3 76.01,7 74.01,9
  pour Bottom (isolate 0.406, rank 6): 74.01,9 21.01,9 20.01,8 20.01,2 18.01,0 4.01,0 0.01,4 0.01,86 5.01,91 18.01,91 20.01,89 20.01,83 22.01,81 74.01,81 76.01,83 76.01,88 78.01,90 93.01,90 96.01,87 96.01,3 93.01,0 79.01,0 76.01,3 76.01,7
GND_HV  (via drill 0.9)
  Top 0.254: 35.41,22.55 C10.2 | U4.6 36.26,22.55 36.26,22.75
  Top 1.5: v14.01,27 14.01,41.5 12.96,42.55 JP1.22 JP1.21
  Bottom 1.5: v26.51,27 v14.01,27
  pour Top (isolate 0.254, rank 2): 21.76,30 29.26,30 29.26,25.5 36.76,25.5 36.76,22.5 21.76,22.5
HV  (via drill 0.35)
  Top 0.254: U$7.6 17.71,37.7 v16.51,36.5 16.33,36.33 R19.1
  Top 1.5: JP1.18 JP1.17 5.88,47.62 4.26,46 4.26,18 5.56,16.7 15.04,16.7 16.29,17.95 16.29,30.95 R19.1
  Bottom 0.254: v16.51,36.5 30.51,36.5 34.01,40 55.01,40 71.01,56 75.01,56 77.01,58 R30.2
N$1
  Top 0.254: U4.4 38.41,24.9 38.01,25.3 38.01,27 | R12.2 39.51,27 38.01,27 | C7.1 38.01,27
N$2  (via drill 0.35)
  Top 0.305: R5.1 v46.01,77 R7.2 | v33.01,77 R6.2 | v25.01,78 22.26,78 | 22.26,78 U2.3 | TP7.TP 19.01,80 21.01,80 22.26,78.75 22.26,78
  Bottom 0.305: v46.01,77 v33.01,77 26.01,77 v25.01,78
N$3  (via drill 0.35)
  Top 0.305: R7.1 38.58,76 v37.01,76 | U2.1 24.96,76.05 v25.01,76 25.01,75 26.01,74 R10.2
  Bottom 0.305: v37.01,76 v25.01,76
N$4  (via drill 0.35)
  Top 0.305: Q2.3 v24.01,70 | v33.01,70 32.01,71 R9.1 | Q1.4 49.03,70 v44.01,70 43.01,69 TP9.TP
  Bottom 0.305: v24.01,70 v33.01,70 v44.01,70
N$5
  Top 3: C20.+ C19.-
N$6
  Top 0.254: U1.9 | U1.9 C2.1 C1.1
N$7
  Top 0.254: C1.2 49.18,52.73 R1.2
N$8
  Top 0.254: U1.2 L1.P$1 | L1.P$1 | TP3.TP L1.P$1
N$9
  Top 0.305: R31.2 15.83,74.08 17.22,75.47 U3.1 17.86,76.35 19.46,77.95 U2.4 19.26,78.5 17.51,78.5 TP8.TP
N$10
  Top 0.254: U1.8 44.51,54.15 U1.1 44.51,58.47 TP1.TP
  Top 1.5: R11.1 46.04,60 44.51,58.47
N$11
  Top 0.254: U1.5 39.04,55.15 | 39.04,55.15 R3.1 | 39.04,55.15 39.03,55.15 | 39.03,55.15 R2.2 | TP4.TP 36.96,55.15 39.03,55.15
N$12
  Top 0.254: 33.29,50.18 C5.2 | U1.6 40.9,54.65 L1.P$2 | L1.P$2 40.9,51.08 R3.2 | L1.P$2 40.9,49.16 C4.1 | R4.2 26.56,44.55 21.66,39.65 U$7.3 | TP2.TP 33.51,46.77 33.51,48.5
  pour Top (isolate 0.254): 41.51,52 41.51,48.25 25.01,48.25 25.01,52
N$13  (via drill 0.35)
  Top 0.305: Q2.1 17.06,70.95 | 17.06,70.95 v17.01,71 | v34.01,71 34.01,73 33.01,74 R10.1 | TP10.TP 16.01,69.9 17.06,70.95
  Bottom 0.305: v17.01,71 v34.01,71
N$14
  Top 0.254: R12.1 39.43,30 C6.1
N$15
  Top 3: C19.+ C18.-
N$16
  Top 0.254: R13.2 42.01,27 41.51,26.5 41.51,25.75 41.26,25.5 39.26,25.5 39.01,25.25 U4.3
N$17
  Top 0.254: U4.1 40.36,23.75 45.18,23.75 R14.2
N$18
  Top 0.254: U4.12 39.61,15.25 41.26,15.25
  pour Top (isolate 0.305, rank 2): 39.01,17.25 39.01,13.75 62.01,13.75 62.01,29.5 55.26,29.5 55.26,17.25
N$19
  Top 0.254: U4.10 38.41,19.65 38.26,19.5 37.76,19.5 37.51,19.25 37.51,16.45 C8.1
N$20
  Top 0.254: U4.13 40.86,20.4 41.01,20.25 41.01,18.8 C9.2
N$21
  Top 0.254: 43.01,18.8 C9.1 | L2.P$2 48.26,20 | U4.7 41.76,22
  pour Top (isolate 0.254): 42.26,17.25 50.51,17.25 50.51,23.25 41.01,23.25 41.01,21 42.26,21
N$22
  Top 0.254: 35.41,21.45 C10.1 | 26.66,21.05 Q3.3 | 29.83,18.59 R18.2 | 32.53,18.42 C13.1 | U4.8 36.51,21.45 36.51,21.5
  pour Top (isolate 0.305): 36.01,17 25.01,17 25.01,22 37.01,22 37.01,21 37.01,17
N$23  (via drill 0.35)
  Top 0.254: 20.51,22.48 Q3.5 | C14.1 20.43,24.13 | R16.2 29.43,31 v28.26,31 | U$7.5 20.66,38.35 21.01,38 v21.01,31
  Bottom 0.254: v28.26,31 v21.01,31
  pour Top (isolate 0.254): 18.26,16.75 21.76,16.75 21.76,33.25 18.26,33.25
N$24
  Top 0.254: U4.5 37.81,24.7 37.01,25.5 33.51,25.5 33.01,26 R17.2 R16.1
N$25
  Top 3: C18.+ C17.-
N$26
  pour Top (isolate 0.305): 48.01,66 76.51,66 76.51,32.5 69.51,32.5 69.51,62 48.01,62
N$27
  Top 0.254: 29.93,15.5 R18.1 | R18.1 32.53,15.58 C13.2 36.06,16.05 36.51,16.5 36.51,19.75 37.16,20.4 U4.9 | R18.1 25.43,15.58 23.51,17.5 23.51,21.25 24.66,22.41 Q3.4
N$28
  Bottom 0.254: R21.1 R22.2 71.26,66.83 71.26,70 72.76,71.5 77.76,71.5 81.26,68 82.01,68 83.51,66.5 83.51,63.82 JP2.7
N$29
  Top 1.5: D1.C 76.53,24.42 R20.1
N$30  (via drill 0.35)
  Top 0.254: v77.01,46.5 79.51,46.5 80.01,46 82.51,46 83.51,47 83.51,61.91 JP2.5
  Bottom 0.254: R25.2 R27.1 76.83,46.5 v77.01,46.5
N$31
  Bottom 0.254: R28.1 65.26,62.67 65.26,64.83 | 65.26,65 65.26,64.83 | 65.26,64.83 R23.2 67.01,66.58 67.01,70.5 68.51,72 78.51,72 82.01,68.5 83.76,68.5 85.58,66.67 JP2.3
N$32
  Bottom 0.254: JP2.9 82.45,59.05 79.76,61.75 79.76,68.68 77.44,71 76.01,71 75.26,70.25 75.26,66.83 R24.2 R29.1
N$33
  Bottom 0.254: R26.2 R30.1 78.08,62.42 82.01,58.5 83.75,58.5 JP2.11
N$100  (via drill 0.35)
  Top 0.254: U$7.9 28.21,37.7 v30.01,39.5 | v30.01,62.5 30.01,64.58 R8.1
  Top 0.305: R8.1 31.01,65 31.01,67.58 R9.2 24.86,71 U2.5 18.68,74.92 R31.1 | Q1.2 Q1.1 | Q1.2 Q1.3 | TP5.TP 47.01,67 50.01,67 51.64,68.64 Q1.2
  Top 3: 50.51,73.5 42.41,73.5 33.91,65 31.01,65
  Bottom 0.254: v30.01,39.5 30.01,49.38 29.98,49.85 29.98,50.62 30.01,51.09 v30.01,62.5
  pour Top: 50.01,68 54.01,68 54.01,78.5 50.01,78.5
PREREG  (via drill 0.35)
  Top 0.305: 57.01,60 R11.2
  Bottom 0.254: R28.2 64.93,59.5 v61.51,59.5
  pour Top (isolate 0.406, rank 3): 69.01,32 83.51,32 83.51,28 55.01,28 55.01,62.5 69.01,62.5
V_BATT  (via drill 0.35)
  Top 0.254: R8.2 28.51,64.08 v28.51,62.5 | U$7.10 27.36,38.35 v28.51,39.5 30.01,41 v31.01,41
  Top 0.305: 27.01,65 R8.2
  Top 1: JP1.9 JP1.11 JP1.12 10.8,56 JP1.10 JP1.9
  Top 2.54: 10.8,56 9.8,57 9.01,57
  Top 3: 10.8,56 11.2,56.4 14.11,56.4 22.71,65 27.01,65
  Bottom 0.254: v28.51,62.5 v28.51,39.5 | v31.01,41 53.51,41 69.01,56.5 R21.2
V_USB  (1 unrouted)
(copper drawn outside any net)
  shapes: Top area x2

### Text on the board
tPlace: ZIPTIE NOTCH | BATTERY VOLTAGE / CUTOFF | 3.3V | CURRENT SENSE | BACKUP POWER | 12V | BOARD # / 1 2 3 4 | REV C | PWR
bPlace: PREREG | BAT | 3.3 | 12.0 | CAP
tNames: U7
Notes: Indicator LEDs should be placed in the bottom corners, filling the avaliable space from left to right | If possible, connect the 3v3 pins on either side on every module | RF Connectors should go in this notch | Debug connectors should go in this notch

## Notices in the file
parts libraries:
SparkFun-PowerSymbols: Licensing: Creative Commons ShareAlike 4.0 International - https://creativecommons.org/licenses/by-sa/4.0
